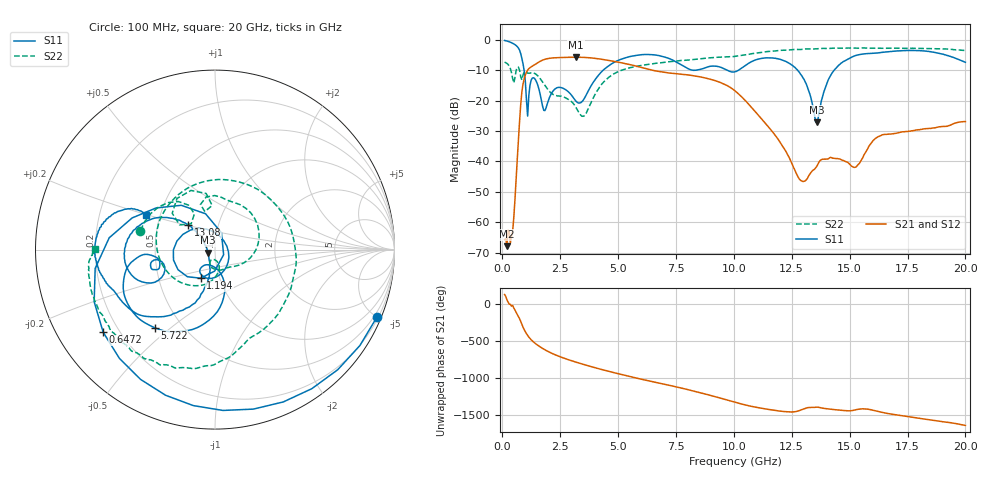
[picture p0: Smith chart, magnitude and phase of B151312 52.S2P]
!  2-Port S-parameters saved by WinCal
! VAR MeasName=S-Parameters (CALIBRATED_DATA) read from VNA (N5244A)
! VAR MeasDate=12/8/2015 5:47:51 PM
! VAR NAME=B151312 52
! VAR FILENAME=B151312 52.S2P
! VAR DATE=12/8/2015 5:47:51 PM
! VAR PHYS_PORTS=1,2
# Hz S DB R 50
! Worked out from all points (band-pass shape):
!   401 points, 100 MHz to 20 GHz, reference 50 ohm
!   highest |S21| = -5.71 dB at 3.184 GHz (marker M1); lowest = -67.9 dB at 199.5 MHz (marker M2)
!   |S21| within 3 dB of the highest: 1.284 GHz to 5.819 GHz (4.535 GHz wide, 128 % of centre)
!   lowest |S11| = -27.2 dB at 13.58 GHz (marker M3), VSWR 1.09, Z = 46.1 - j1.51 ohm
!   |S11| at or under -10 dB: 942.2 MHz to 4.354 GHz (3.412 GHz wide, 129 % of centre); 9.714 GHz to 10.2 GHz (484.4 MHz wide, 4.87 % of centre); 12.76 GHz to 14.33 GHz (1.573 GHz wide, 11.6 % of centre)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
!   |S22| runs from -25.1 to -2.7 dB; largest |S21 - S12| = 0.002
!   S11 on the Smith chart (normalised r, x): 100 MHz: 0.29, -4.99; 647.2 MHz: 0.14, -0.32; 1.194 GHz: 0.81, -0.27; 5.722 GHz: 0.35, -0.44; 13.08 GHz: 0.71, +0.20; 20 GHz: 0.42, +0.20
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1e8  -0.20 -22.6  -65.69 126.4  -66.02 124.9  -7.35 165.6
1.995e8  -0.38 -44.4  -67.85 55.3  -68.71 52.2  -7.74 150.7
4.4825e8  -1.13 -97.9  -62.90 -21.0  -63.17 -24.6  -12.76 119.9
6.4725e8  -2.22 -143.5  -39.17 -141.1  -39.15 -141.4  -8.99 126.6
8.96e8  -7.91 144.8  -14.48 47.0  -14.49 47.0  -11.56 107.8
1.1945e9  -14.97 -116.8  -9.16 -104.5  -9.16 -104.5  -10.94 66.7
1.54275e9  -15.15 141.5  -7.45 161.2  -7.45 161.1  -11.90 14.6
1.94075e9  -21.08 -28.6  -6.20 85.7  -6.20 85.7  -16.06 -33.7
2.488e9  -15.64 -109.0  -5.82 10.0  -5.82 10.0  -18.53 -70.1
3.1845e9  -20.19 -120.3  -5.71 -63.6  -5.71 -63.6  -22.27 -110.9
3.43325e9  -20.37 -94.5  -5.75 -87.2  -5.74 -87.2  -25.09 -104.5
4.42825e9  -9.51 -86.5  -6.54 -173.7  -6.54 -173.6  -13.49 -110.2
5.72175e9  -5.19 -127.7  -8.52 87.0  -8.49 87.1  -8.85 132.7
6.7665e9  -5.18 -158.2  -10.40 14.9  -10.40 14.7  -7.62 43.9
8.20925e9  -9.97 -169.7  -11.75 -88.5  -11.73 -88.6  -6.46 -27.4
1.005e10  -10.48 -159.2  -16.76 116.5  -16.74 116.4  -5.43 -70.1
1.308475e10  -13.85 137.8  -46.37 33.0  -46.40 32.5  -3.00 -114.6
1.338325e10  -20.77 142.5  -43.10 48.4  -43.14 48.0  -2.99 -117.6
1.358225e10  -27.16 -158.1  -41.61 51.2  -41.65 51.0  -2.92 -120.7
1.45275e10  -8.35 -117.9  -39.13 11.7  -39.13 11.4  -2.76 -130.8
1.67165e10  -3.89 -165.1  -31.02 -38.7  -30.95 -39.1  -2.72 -151.9
2e10  -7.37 153.4  -26.88 164.5  -27.01 164.1  -3.49 179.6
